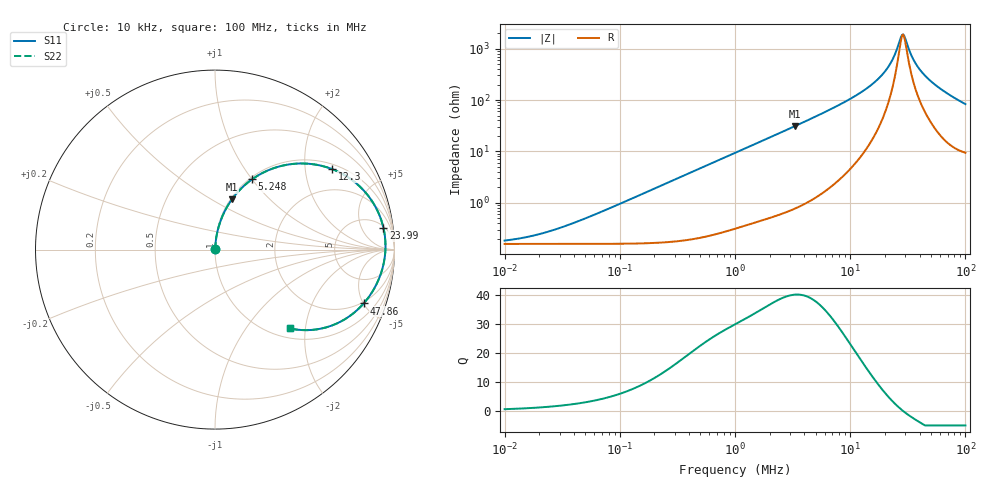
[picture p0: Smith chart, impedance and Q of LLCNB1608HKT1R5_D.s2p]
! LLCNB1608HKT1R5_D  S-PARAMETER MODEL  ( Standard Model )
! Model Generated by TAIYO YUDEN Corporation (http://www.ty-top.com)
! Version 1.0
! TAIYO YUDEN Control No. 200410
! Copyright(c) 2020 TAIYO YUDEN CO.,LTD. All Rights Reserved.
! Product Description (link to TY-COMPAS)
! https://ds.yuden.co.jp/TYCOMPAS/or/detail?pn=LLCNB1608HKT1R5MD&u=M
! Products Name : Inductors
! Characteristics :
!  Inductance : 1.5 [uH] , SRF(min) : - [Hz] , DC Resistance(max) : 200 [mOhm]
!  Rated Current : Saturation  1.7 [A] (dL = 30 [%]), Temp Rise  1.3 [A] (dT = 40 [degC])
!  Case Size : 1.6 x 0.8 / 0.063 x 0.031 [mm/inch] , Thickness : 0.8 / 0.031 [mm/inch]
!  (Conditions: Temperature = 25 [degC] , DC Bias Current = 0 [A])
! External Node Assignments :
!  1  o---GGG---o  2
! GND o---------o GND
! Frequency Range : 10kHz  -  100MHz  [ 402 STEP ]
# MHz S RI R 50
! Freq[MHz].  S11 Real  S11 Imag  S21 Real  S21 Imag  S12 Real  S12 Imag  S22 Real  S22 Imag
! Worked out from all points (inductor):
!   401 points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, 10 kHz to 100 MHz, reference 50 ohm
!   read as one part in series: L = 1.51 uH near 51.29 kHz
!   highest Q = 40 at 3.311 MHz (marker M1), where L = 1.49 uH
!   self-resonance near 28.74 MHz
!   S11 on the Smith chart (normalised r, x): 10 kHz: 1.00, +0.00; 5.248 MHz: 1.03, +1.00; 12.3 MHz: 1.16, +2.78; 23.99 MHz: 6, +13; 47.86 MHz: 1.87, -5.02; 100 MHz: 1.19, -1.65
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0.01  0.0016 0.000943  0.9984 -0.000943  0.9984 -0.000943  0.0016 0.000943
0.020893  0.0016 0.00197  0.9984 -0.00197  0.9984 -0.00197  0.0016 0.00197
0.046774  0.00162 0.00441  0.9984 -0.00441  0.9984 -0.00441  0.00162 0.00441
0.218776  0.00211 0.0206  0.9979 -0.0206  0.9979 -0.0206  0.00211 0.0206
1  0.0118 0.0925  0.9882 -0.0925  0.9882 -0.0925  0.0118 0.0925
3.311311  0.0938 0.2794  0.9062 -0.2794  0.9062 -0.2794  0.0938 0.2794
4.677351  0.1712 0.3639  0.8288 -0.3639  0.8288 -0.3639  0.1712 0.3639
5.248075  0.2075 0.3923  0.7925 -0.3923  0.7925 -0.3923  0.2075 0.3923
8.51138  0.429 0.4768  0.571 -0.4768  0.571 -0.4768  0.429 0.4768
12.30269  0.6517 0.449  0.3483 -0.449  0.3483 -0.449  0.6517 0.449
17.37801  0.8402 0.3165  0.1598 -0.3165  0.1598 -0.3165  0.8402 0.3165
21.87762  0.9205 0.181  0.0795 -0.181  0.0795 -0.181  0.9205 0.181
23.98833  0.9386 0.1208  0.0614 -0.1208  0.0614 -0.1208  0.9386 0.1208
27.54229  0.9499 0.0284  0.0501 -0.0284  0.0501 -0.0284  0.9499 0.0284
28.84032  0.9494 -0.00228  0.0506 0.00228  0.0506 0.00228  0.9494 -0.00228
30.19952  0.947 -0.0327  0.053 0.0327  0.053 0.0327  0.947 -0.0327
33.88442  0.9327 -0.1065  0.0673 0.1065  0.0673 0.1065  0.9327 -0.1065
37.15352  0.9134 -0.1628  0.0866 0.1628  0.0866 0.1628  0.9134 -0.1628
41.68694  0.8803 -0.2286  0.1197 0.2286  0.1197 0.2286  0.8803 -0.2286
47.86301  0.8283 -0.3001  0.1717 0.3001  0.1717 0.3001  0.8283 -0.3001
69.1831  0.6331 -0.4292  0.3669 0.4292  0.3669 0.4292  0.6331 -0.4292
100  0.4183 -0.4395  0.5817 0.4395  0.5817 0.4395  0.4183 -0.4395
